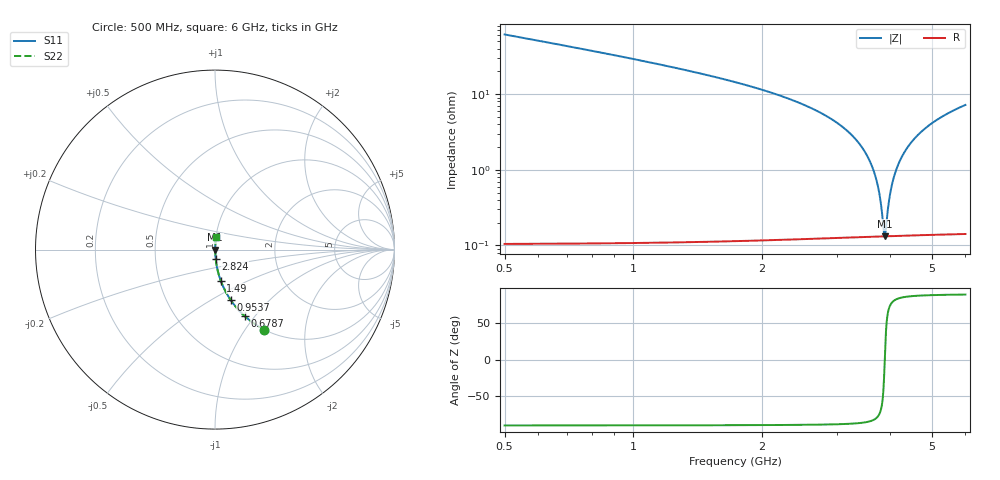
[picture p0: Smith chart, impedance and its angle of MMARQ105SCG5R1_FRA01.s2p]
! MMARQ105SCG5R1_FRA01  S-PARAMETER MODEL  ( General Type )
! Model Generated by TAIYO YUDEN Corporation (http://www.ty-top.com)
! Version 1.0
! TAIYO YUDEN Control No. 200326
! Copyright(c) 2020 TAIYO YUDEN CO.,LTD. All Rights Reserved.
! Product Description (link to TY-COMPAS)
! https://ds.yuden.co.jp/TYCOMPAS/or/detail?pn=MMARQ105SCG5R1CFRA01&u=M
! Products Name : Multilayer Ceramic Capacitors
! Characteristics :
!  Capacitance : 5.1 pF , Rated Voltage : 250V , TCC : CG / C0G
!  Case Size : 1.0 x 0.5 / 0.039 x 0.02 [mm/inch] , Thickness : 0.5 / 0.02 [mm/inch]
!  (Conditions: Temperature = 25 degC , DC Bias Current/Voltage = 0A / 0V)
! External Node Assignments :
!  1  o---| |---o  2
! GND o---------o GND
! Frequency Range : 500MHz  -  6GHz  [ 401 STEP ]
# MHz S RI R 50
! Freq[MHz].  S11 Real  S11 Imag  S21 Real  S21 Imag  S12 Real  S12 Imag  S22 Real  S22 Imag
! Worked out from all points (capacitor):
!   401 points, 500 MHz to 6 GHz, reference 50 ohm
!   read as one part in series: C = 5.1 pF near 527.5 MHz
!   lowest |Z| = 132 mohm at 3.882 GHz (marker M1)
!   series resonance near 3.884 GHz, so ESL is about 330 pH
!   S11 on the Smith chart (normalised r, x): 500 MHz: 1.00, -1.23; 678.8 MHz: 1.00, -0.89; 953.8 MHz: 1.00, -0.61; 1.49 GHz: 1.00, -0.36; 2.824 GHz: 1.00, -0.10; 6 GHz: 1.00, +0.14
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500  0.274 -0.4452  0.726 0.4452  0.726 0.4452  0.274 -0.4452
678.75  0.1664 -0.3712  0.8336 0.3712  0.8336 0.3712  0.1664 -0.3712
953.75  0.0872 -0.2804  0.9128 0.2804  0.9128 0.2804  0.0872 -0.2804
1421.25  0.0359 -0.1831  0.9641 0.1831  0.9641 0.1831  0.0359 -0.1831
1490  0.0319 -0.1727  0.9681 0.1727  0.9681 0.1727  0.0319 -0.1727
2342.5  0.00829 -0.0839  0.9917 0.0839  0.9917 0.0839  0.00829 -0.0839
2823.75  0.00393 -0.0518  0.9961 0.0518  0.9961 0.0518  0.00393 -0.0518
3250  0.0021 -0.0287  0.9979 0.0287  0.9979 0.0287  0.0021 -0.0287
3497.5  0.00158 -0.0168  0.9984 0.0168  0.9984 0.0168  0.00158 -0.0168
3662.5  0.00139 -0.00941  0.9986 0.00941  0.9986 0.00941  0.00139 -0.00941
3772.5  0.00133 -0.00467  0.9987 0.00467  0.9987 0.00467  0.00133 -0.00467
3855  0.00132 -0.00121  0.9987 0.00121  0.9987 0.00121  0.00132 -0.00121
3882.5  0.00132 -7.03e-05  0.9987 7.03e-05  0.9987 7.03e-05  0.00132 -7.03e-05
3910  0.00132 0.00106  0.9987 -0.00106  0.9987 -0.00106  0.00132 0.00106
3965  0.00134 0.00329  0.9987 -0.00329  0.9987 -0.00329  0.00134 0.00329
4020  0.00136 0.0055  0.9986 -0.0055  0.9986 -0.0055  0.00136 0.0055
4088.75  0.0014 0.00821  0.9986 -0.00821  0.9986 -0.00821  0.0014 0.00821
4171.25  0.00147 0.0114  0.9985 -0.0114  0.9985 -0.0114  0.00147 0.0114
4322.5  0.00164 0.0171  0.9984 -0.0171  0.9984 -0.0171  0.00164 0.0171
4528.75  0.00196 0.0246  0.998 -0.0246  0.998 -0.0246  0.00196 0.0246
5092.5  0.0033 0.0438  0.9967 -0.0438  0.9967 -0.0438  0.0033 0.0438
6000  0.00654 0.0714  0.9935 -0.0714  0.9935 -0.0714  0.00654 0.0714
